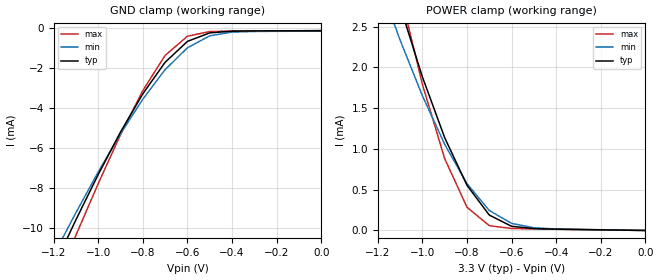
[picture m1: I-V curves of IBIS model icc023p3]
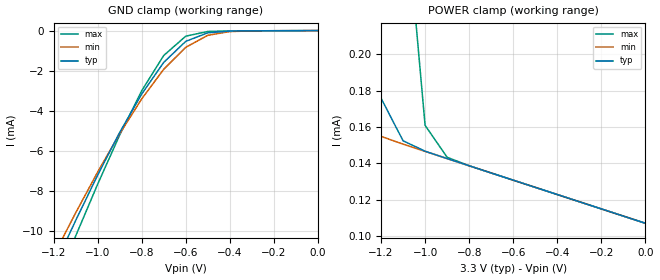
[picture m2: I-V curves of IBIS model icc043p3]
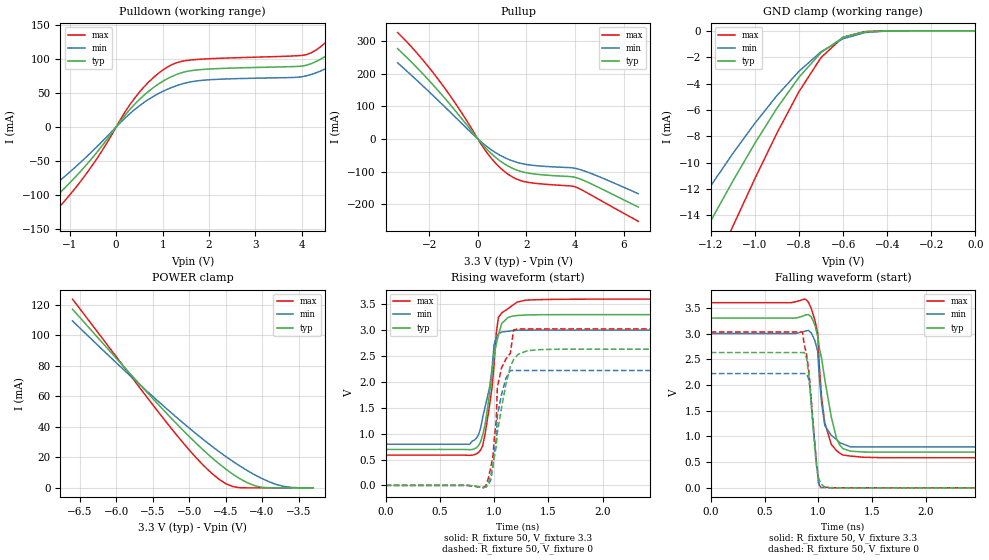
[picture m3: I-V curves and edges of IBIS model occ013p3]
[IBIS ver]   2.1
[File name]   mpc9774.ibs
[File Rev]   2.2 {April 29, 2002}
[Date]   December 20th, 2002
[Disclaimer]   This information is for modeling purposes only
|   and is not guaranteed.
[Source]   Timing Solutions Operations
[Copyright]   Copyright 2001, Motorola Incorporated,
|   all rights reserved.
| Component MPC9774 for 3.3V Application!
[Component]   MPC97743p3
[Manufacturer]   Motorola
[Package]
|   typ   min   max
R_pkg   0.048   .038   0.053
L_pkg   6.045nH   5.084nH   7.950nH
C_pkg   0.813pF   0.560pF   1.157pF
[Pin]   signal_name   model_name   R_pin   L_pin   C_pin
2   MRB/OE   icc023p3   0.04   0.35nH   0.053pF
3   CLKB_STOP   icc023p3   0.04   0.35nH   0.053pF
4   FSEL_B   icc043p3   0.04   0.35nH   0.053pF
5   FSEL_C   icc043p3   0.04   0.35nH   0.053pF
6   PLL_EN   icc023p3   0.04   0.35nH   0.053pF
7   FSEL_A   icc043p3   0.04   0.35nH   0.053pF
8   CCLK_SEL   icc043p3   0.04   0.35nH   0.053pF
9   CCLK0   icc043p3   0.04   0.35nH   0.053pF
10   CCLK1   icc023p3   0.04   0.35nH   0.053pF
14   FSEL_FB0   icc043p3   0.04   0.35nH   0.053pF
16   QA4   occ013p3   0.04   0.35nH   0.053pF
18   QA3   occ013p3   0.04   0.35nH   0.053pF
20   FSEL_FB1   icc043p3   0.04   0.35nH   0.053pF
21   QA2   occ013p3   0.04   0.35nH   0.053pF
23   QA1   occ013p3   0.04   0.35nH   0.053pF
25   QA0   occ013p3   0.04   0.35nH   0.053pF
29   QFB   icc023p3   0.04   0.35nH   0.053pF
31   FB_IN   icc023p3   0.04   0.35nH   0.053pF
32   QB4   occ013p3   0.04   0.35nH   0.053pF
34   QB3   occ013p3   0.04   0.35nH   0.053pF
36   QB2   occ013p3   0.04   0.35nH   0.053pF
38   QB1   occ013p3   0.04   0.35nH   0.053pF
40   QB0   occ013p3   0.04   0.35nH   0.053pF
44   QC3   occ013p3   0.04   0.35nH   0.053pF
46   QC2   occ013p3   0.04   0.35nH   0.053pF
48   QC1   occ013p3   0.04   0.35nH   0.053pF
50   QC0   occ013p3   0.04   0.35nH   0.053pF
52   VC0_SEL   icc043p3   0.04   0.35nH   0.053pF
|Component Inputs and Outputs at 2.5V Application
[Component]   MPC97742p5
[Manufacturer]   Motorola
[Package]
|   typ   min   max
R_pkg   0.048   .038   0.053
L_pkg   6.045nH   5.084nH   7.950nH
C_pkg   0.813pF   0.560pF   1.157pF
[Pin]   signal_name   model_name   R_pin   L_pin   C_pin
2   MRB/OE   icc022p5   0.04   0.35nH   0.053pF
3   CLKB_STOP   icc022p5   0.04   0.35nH   0.053pF
4   FSEL_B   icc042p5   0.04   0.35nH   0.053pF
5   FSEL_C   icc042p5   0.04   0.35nH   0.053pF
6   PLL_EN   icc022p5   0.04   0.35nH   0.053pF
7   FSEL_A   icc042p5   0.04   0.35nH   0.053pF
8   CCLK_SEL   icc042p5   0.04   0.35nH   0.053pF
9   CCLK0   icc042p5   0.04   0.35nH   0.053pF
10   CCLK1   icc022p5   0.04   0.35nH   0.053pF
14   FSEL_FB0   icc042p5   0.04   0.35nH   0.053pF
16   QA4   occ012p5   0.04   0.35nH   0.053pF
18   QA3   occ012p5   0.04   0.35nH   0.053pF
20   FSEL_FB1   icc042p5   0.04   0.35nH   0.053pF
21   QA2   occ012p5   0.04   0.35nH   0.053pF
23   QA1   occ012p5   0.04   0.35nH   0.053pF
25   QA0   occ012p5   0.04   0.35nH   0.053pF
29   QFB   icc022p5   0.04   0.35nH   0.053pF
31   FB_IN   icc022p5   0.04   0.35nH   0.053pF
32   QB4   occ012p5   0.04   0.35nH   0.053pF
34   QB3   occ012p5   0.04   0.35nH   0.053pF
36   QB2   occ012p5   0.04   0.35nH   0.053pF
38   QB1   occ012p5   0.04   0.35nH   0.053pF
40   QB0   occ012p5   0.04   0.35nH   0.053pF
44   QC3   occ012p5   0.04   0.35nH   0.053pF
46   QC2   occ012p5   0.04   0.35nH   0.053pF
48   QC1   occ012p5   0.04   0.35nH   0.053pF
50   QC0   occ012p5   0.04   0.35nH   0.053pF
52   VC0_SEL   icc042p5   0.04   0.35nH   0.053pF
| Models and submodels in the file (6): icc023p3 (Input), icc043p3 (Input), occ013p3 (Output), occ012p5 (Output), icc042p5 (Input), icc022p5 (Input)
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|This is a Model of an Input with a 25,000 ohm Pull_up at 3.3V
[Model]   icc023p3
Model_type   Input
Polarity   Non-Inverting
Vmeas=1.5
Vinl=0.8
Vinh=2.0
|Variable   typ   min   max
C_comp   5p   5p   5p
[Temperature Range]   27.00   100.00   -45.00
[Power Clamp Reference]   3.30V   3.00V   3.60V
[Gnd Clamp Reference]   0.000V   0.000V   0.000V
[Voltage Range]   3.30V   3.00V   3.60V
[Pulldown Reference]   0.000V   0.000V   0.000V
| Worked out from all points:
|   GND clamp passes 1 mA (typ) near -0.63 V on its own axis
|   POWER clamp passes 1 mA (typ) near -0.88 V on its own axis
[GND_clamp]
| voltage   I(typ)   I(min)   I(max)
-3.3V     -65.56mA   -61.83mA   -70.36mA
-1.2V     -11.94mA   -11.35mA   -13.02mA
-1.1V     -9.583mA   -9.224mA   -10.36mA
-1V       -7.318mA   -7.188mA   -7.771mA
-900mV    -5.193mA   -5.279mA   -5.323mA
-800mV    -3.28mA    -3.546mA   -3.115mA
-700mV    -1.702mA   -2.069mA   -1.359mA
-600mV    -655uA     -975.9uA   -396.7uA
-500mV    -229.7uA   -377.6uA   -163.2uA
-400mV    -143.9uA   -192.2uA   -135.8uA
1.97fV    -118.8uA   -142.6uA   -118.8uA
[POWER_clamp]
| voltage   I(typ)  I(min)  I(max)
-3.3V     32.89mA    26.85mA    40.63mA
-1.2V     3.727mA    3.095mA    4.229mA
-1.1V     2.756mA    2.338mA    2.93mA
-1V       1.886mA    1.654mA    1.795mA
-900mV    1.14mA     1.058mA    882.5uA
-800mV    554.8uA    575uA      285.5uA
-700mV    189.3uA    245.4uA    59.28uA
-600mV    51.31uA    86.95uA    24.32uA
-500mV    23.2uA     32.54uA    18.63uA
-400mV    16.45uA    18.02uA    14.85uA
0V        148.9pA    557.5pA    4.024pA
|This model is an Input with a 25,000 ohm Pull_down at 3.3V
[Model]   icc043p3
Model_type   Input
Vref=1.5V
Vinl=0.8V
Vinh=2.0V
| Variable   typ   min   max
C_comp   5p   5p   5p
[Temperature Range]   27.00   100.00   -45.00
[Power Clamp Reference]   3.30V   3.00V   3.60V
[Gnd Clamp Reference]   0.000V   0.000V   0.000V
[Voltage Range]   3.30V   3.00V   3.60V
[Pulldown Reference]   0.000V   0.000V   0.000V
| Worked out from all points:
|   GND clamp passes 1 mA (typ) near -0.64 V on its own axis
|   POWER clamp passes 1 mA (typ) near -1.44 V on its own axis
[GND_clamp]
| voltage   I(typ)   I(min)   I(max)
-3.3V     -65.45mA   -61.69mA   -70.25mA
-1.2V     -11.83mA   -11.21mA   -12.91mA
-1.1V     -9.467mA   -9.084mA   -10.24mA
-1V       -7.201mA   -7.048mA   -7.655mA
-900mV    -5.077mA   -5.139mA   -5.207mA
-800mV    -3.163mA   -3.405mA   -2.998mA
-700mV    -1.585mA   -1.928mA   -1.242mA
-600mV    -537uA     -834.6uA   -278.5uA
-500mV    -111.2uA   -235.5uA   -44.5uA
-400mV    -25.07uA   -49.72uA   -17.01uA
1.97fV    -61.68pA   -9.69nA    -3.014pA
[POWER_clamp]
| voltage   I(typ)  I(min)  I(max)
-3.3V     27.21mA    21.56mA    34.07mA
-1.5V     1.4mA      337.1uA    3.859mA
-1.4V     717.9uA    194.4uA    2.632mA
-1.3V     311.6uA    162.1uA    1.579mA
-1.2V     175.9uA    154.8uA    767.8uA
-1.1V     152.4uA    150.5uA    297.2uA
-1V       146.6uA    146.5uA    160.9uA
-900mV    142.6uA    142.6uA    143.3uA
-800mV    138.6uA    138.6uA    138.6uA
1.97fV    106.9uA    106.9uA    106.9uA
|  Output Buffer at 3.3V Application
[Model]   occ013p3
Model_type   Output
Enable   Active-Low
Polarity   Non-Inverting
Vref=1.5
Rref=50
Cref=1pf
| Variable   typ   min   max
C_comp   5p   5p   5p
[Temperature Range]   27.00   100.00   -45.00
[Voltage Range]   3.30V   3.00V   3.60V
[Pulldown Reference]   0.000V   0.000V   0.000V
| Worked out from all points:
|   slope of the pulldown table from 0 to 0.495 V, typ, clamps not added: 12.4 ohm
|   slope of the pullup table from 0 to 0.495 V, typ, clamps not added: 12.1 ohm
|   GND clamp passes 1 mA (typ) near -0.64 V on its own axis
|   POWER clamp passes 1 mA (typ) near -4.06 V on its own axis
|   rising waveform, R_fixture 50, V_fixture 3.3: 20-80 % time 105ps typ, 105ps min, 91.8ps max; typ from 0.695 V to 3.3 V
|   falling waveform, R_fixture 50, V_fixture 3.3: 20-80 % time 133ps typ, 61.6ps min, 76.5ps max; typ from 3.3 V to 0.695 V
|   rising waveform, R_fixture 50, V_fixture 0: 20-80 % time 127ps typ, 77.6ps min, 112ps max; typ from 0 V to 2.63 V
|   falling waveform, R_fixture 50, V_fixture 0: 20-80 % time 63.4ps typ, 54ps min, 76.3ps max; typ from 2.63 V to 0 V
[Pulldown]
|voltage   I(typ)   I(min)   I(max)
-3.3V     -209.8mA   -184.1mA   -233.1mA
-2.5V     -171.4mA   -145.7mA   -196.3mA
-2V       -144.6mA   -120.9mA   -169.9mA
-1.6V     -121.3mA   -100.1mA   -144.4mA
-600mV    -52.28mA   -41.26mA   -64.61mA
500mV     40.26mA    30.94mA    50.94mA
1.2V      74.05mA    58.02mA    91.38mA
4.1V      90.56mA    75mA       106.1mA
4.8V      118.5mA    95.76mA    145.2mA
5.2V      146.1mA    114.5mA    186.5mA
5.7V      200mA      148.6mA    270.9mA
6.6V      419.9mA    278.5mA    628.6mA
[Pullup]
| voltage  I(typ)   I(min)   I(max)
-3.3V     276.2mA    233mA      325.6mA
-2.5V     217.6mA    178.8mA    262.3mA
-1.7V     153.4mA    122.6mA    189.2mA
-800mV    74.59mA    57.3mA     95.02mA
300mV     -26.06mA   -19.2mA    -34.48mA
700mV     -54.72mA   -40.53mA   -71.91mA
1.1V      -76.73mA   -57.15mA   -100.1mA
1.5V      -92.4mA    -69.23mA   -119.7mA
1.9V      -102.1mA   -76.99mA   -130.5mA
4V        -117.6mA   -89.99mA   -146.7mA
4.8V      -142.5mA   -110mA     -177.7mA
6.6V      -208.6mA   -167.9mA   -252.3mA
[GND_clamp]
| voltage  I(typ)   I(min)   I(max)
-3.3V     -85.27mA   -74.38mA   -97.87mA
-1.4V     -20.76mA   -16.98mA   -26.15mA
-1.3V     -17.56mA   -14.32mA   -22.34mA
-1.2V     -14.43mA   -11.76mA   -18.57mA
-1.1V     -11.4mA    -9.311mA   -14.84mA
-900mV    -5.871mA   -4.914mA   -7.763mA
-800mV    -3.524mA   -3.07mA    -4.613mA
-700mV    -1.653mA   -1.587mA   -2.027mA
-600mV    -494uA     -597.7uA   -480.9uA
-500mV    -78.44uA   -130.1uA   -51.01uA
-400mV    -7.209uA   -15.25uA   -2.718uA
1.97fV    -33.27pA   -701.5pA   -3.87pA
[POWER_clamp]
| voltage
-6.6V     117mA      109.4mA    123.6mA
-5.8V     74.29mA    73.06mA    73.28mA
-5.2V     43.37mA    47.3mA     36.28mA
-4.9V     29.01mA    35.26mA    19.52mA
-4.6V     16.15mA    24.09mA    5.976mA
-4.5V     12.36mA    20.62mA    2.814mA
-4.4V     8.904mA    17.3mA     800.8uA
-4.2V     3.283mA    11.23mA    5.412uA
-4.1V     1.379mA    8.513mA    174.8nA
-3.9V     43.18uA    3.908mA    72.88pA
-3.7V     227.2nA    935.3uA    4.59pA
-3.3V     48.11pA    322.6nA    3.568pA
[Ramp]
dV/dt_r   1.56/105p   1.29/169p   1.81/69.3p
dV/dt_f   1.56/127.4p   1.3/192.1p   1.81/88.1p
R_load = 50
[Rising Waveform]
R_fixture = 50
V_fixture = 3.3
V_fixture_min = 3.0
V_fixture_max = 3.6
|Time   Voltage(typ)  Voltage(min)  Voltage(max)
0s        695mV      795.2mV    585.3mV
776ps     691.2mV    795.2mV    581.3mV
858ps     771.9mV    985.6mV    638mV
895ps     972.8mV    1.315V     766.3mV
958ps     1.778V     1.889V     1.542V
1ns       2.487V     2.722V     2.333V
1.04ns    2.904V     2.926V     3.247V
1.07ns    3.129V     2.965V     3.333V
1.21ns    3.283V     2.998V     3.539V
5ns       3.3V       3V         3.6V
[Falling Waveform]
R_fixture = 50
V_fixture = 3.3
V_fixture_min = 3.0
V_fixture_max = 3.6
|Time   Voltage(typ)  Voltage(min)  Voltage(max)
0s        3.3V       3V         3.6V
908ps     3.368V     3.061V     3.608V
994ps     2.939V     2.654V     3.01V
1.01ns    2.718V     2.137V     2.349V
1.03ns    2.52V      1.654V     1.761V
1.06ns    2.104V     1.21V      1.263V
1.12ns    1.384V     1.023V     846.3mV
1.17ns    950.1mV    937.9mV    721mV
1.23ns    761.7mV    854.5mV    637.3mV
5ns       695mV      795.3mV    585.3mV
[Rising Waveform]
R_fixture = 50
V_fixture = 0
V_fixture_min = 0
V_fixture_max = 0
|Time   Voltage(typ)  Voltage(min)  Voltage(max)
0s        286.8pV    9.073nV    24.07pV
924ps     -30.9mV    -32.03mV   -10.33mV
991ps     416.9mV    374.4mV    591mV
1.02ns    757mV      893.3mV    1.26V
1.03ns    1.015V     1.343V     1.899V
1.11ns    1.961V     2.075V     2.446V
1.15ns    2.296V     2.221V     2.553V
1.18ns    2.432V     2.221V     3.004V
1.43ns    2.625V     2.221V     3.025V
5ns       2.632V     2.221V     3.025V
[Falling Waveform]
R_fixture = 50
V_fixture = 0
V_fixture_min = 0
V_fixture_max = 0
|Time   Voltage(typ)  Voltage(min)  Voltage(max)
0s        2.63V      2.222V     3.03V
853ps     2.63V      2.222V     3.03V
890ps     2.524V     2.217V     2.597V
919ps     2.025V     1.996V     2.099V
966ps     783.7mV    921.9mV    881.6mV
982ps     456.5mV    459.8mV    514.4mV
1ns       209.4mV    107mV      137.6mV
1.02ns    95.09mV    4.92mV     24.83mV
1.1ns     3.325mV    2.05mV     9.039mV
5ns       -11.9uV    304.1nV    11.65uV
